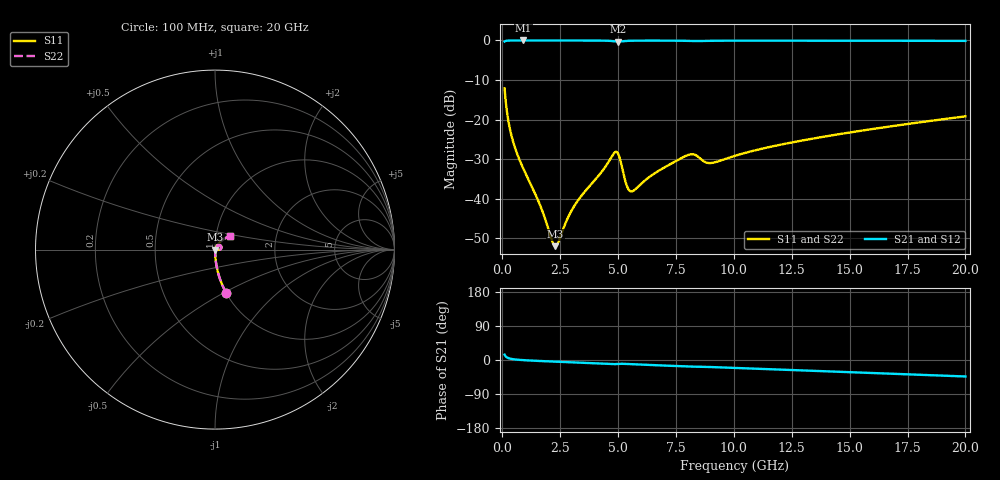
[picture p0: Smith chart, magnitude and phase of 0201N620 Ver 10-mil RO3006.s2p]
# GHz S MA R 50
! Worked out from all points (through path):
!   1601 points, 100 MHz to 20 GHz, reference 50 ohm
!   highest |S21| = -0.02 dB at 908.4 MHz (marker M1); lowest = -0.3 dB at 5 GHz (marker M2)
!   group delay of S21, straight-line fit = 6.21 ps
!   lowest |S11| = -52.0 dB at 2.289 GHz (marker M3), VSWR 1.01, Z = 50.2 - j0.0383 ohm
!   |S11| at or under -10 dB: start of sweep to end of sweep
!   |S22| runs from -52.0 to -12.1 dB; largest |S21 - S12| = 0
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0.1  0.2476 -75.6  0.968 14.1  0.968 14.1  0.2476 -75.6
0.274125  0.09173 -84.6  0.9948 4.7  0.9948 4.7  0.09173 -84.6
0.4109375  0.06029 -86.3  0.9971 2.7  0.9971 2.7  0.06029 -86.3
0.9084375  0.02401 -86.6  0.9981 -0.4  0.9981 -0.4  0.02401 -86.6
1.580062  0.009027 -79.4  0.9979 -2.5  0.9979 -2.5  0.009027 -79.4
2.13975  0.002984 -39.9  0.9975 -4.0  0.9975 -4.0  0.002984 -39.9
2.289  0.002518 -8.7  0.9974 -4.4  0.9974 -4.4  0.002518 -8.7
2.425813  0.002849 19.6  0.9973 -4.7  0.9973 -4.7  0.002849 19.6
2.948187  0.006719 57.9  0.997 -6.0  0.997 -6.0  0.006719 57.9
3.420812  0.01093 64.8  0.9965 -7.1  0.9965 -7.1  0.01093 64.8
4.291437  0.02186 64.4  0.9936 -9.4  0.9936 -9.4  0.02186 64.4
4.813813  0.03733 41.7  0.9767 -10.9  0.9767 -10.9  0.03733 41.7
5.000375  0.0371 14.8  0.9662 -10.4  0.9662 -10.4  0.0371 14.8
5.361063  0.01508 3.8  0.9852 -10.4  0.9852 -10.4  0.01508 3.8
5.547625  0.01239 24.5  0.9897 -11.0  0.9897 -11.0  0.01239 24.5
6.741625  0.02243 60.7  0.9937 -14.1  0.9937 -14.1  0.02243 60.7
8.097312  0.03625 49.8  0.9852 -17.3  0.9852 -17.3  0.03625 49.8
8.9555  0.02821 46.0  0.9873 -18.5  0.9873 -18.5  0.02821 46.0
10.05  0.03486 57.3  0.9921 -21.0  0.9921 -21.0  0.03486 57.3
13.37081  0.05723 55.1  0.9916 -28.5  0.9916 -28.5  0.05723 55.1
16.69162  0.08144 49.1  0.9892 -35.9  0.9892 -35.9  0.08144 49.1
20  0.1098 42.4  0.9857 -43.5  0.9857 -43.5  0.1098 42.4
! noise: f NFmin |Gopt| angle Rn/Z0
0.1  0.0006011  0.9287  0.2312  0.001872
2.301  0.004762  0.8061  4.395  0.005101
4.515  0.0127  0.8539  8.593  0.01844
6.729  0.01247  0.7869  12.77  0.01189
8.943  0.02075  0.8267  16.95  0.02464
11.14  0.0167  0.7451  20.98  0.01274
13.36  0.01835  0.7266  25.02  0.01273
15.57  0.02036  0.7165  29  0.01333
17.79  0.02244  0.7097  32.93  0.01403
20  0.02453  0.7048  36.8  0.01473
